{attribute 'qualified_only'}
{attribute 'strict'}
TYPE eDSP402States :
(
	NOT_READY_TO_SWITCH_ON := 1,
	SWITCH_ON_DISABLED,
	READY_TO_SWITCH_ON,
	SWITCHED_ON,
	OPERATION_ENABLE,
	FAULT,
	QUICK_STOP_ACTIVE
);
END_TYPE
